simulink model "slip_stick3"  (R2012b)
settings: Solver=ode2  StartTime=0.0  StopTime=100  FixedStep=0.001  MaxStep=0.001  RelTol=1e-3
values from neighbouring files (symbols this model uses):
  c = 2200    [coulomb_1.m]    (also in coulomb_10.m = 0.1; coulomb_11.m = 0; coulomb_2.m; coulomb_3.m)
  FG = 500    [coulomb_1.m]    (also in coulomb_10.m = 10; coulomb_11.m = 10; coulomb_2.m; coulomb_3.m)
  FH = 12    [coulomb_10.m]    (also in coulomb_11.m; coulomb_3.m = 600; coulomb_4.m = 600; position_reg_1.m = 3.956)
  k = 10    [coulomb_10.m]    (also in coulomb_11.m; diff_filter_1.m = 250; diff_filter_2.m = 250; dry_friction_1.m = 2200)
  m = 400    [coulomb_1.m]    (also in coulomb_10.m = 10; coulomb_11.m = 10; coulomb_2.m; coulomb_3.m)
  vb = 0.1    [coulomb_10.m]    (also in coulomb_11.m; slip_stick_3.m; slip_stick_31.m; slip_stick_3_1.m)
  vs = 0.05    [position_reg_1.m]    (also in position_reg_2.m; slip_stick_21.m; slip_stick_3.m = 0.01; slip_stick_31.m)
undefined symbols (not defined in the file or in its folder): sgn

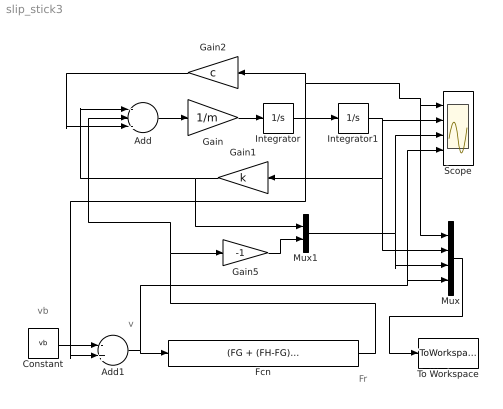
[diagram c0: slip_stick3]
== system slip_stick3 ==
  note: v
  note: vb
  note: Fr
  Add : Sum  Inputs=---
  Add1 : Sum  Inputs=-+
  Constant : Constant  Value=vb
  Fcn : Fcn  Expr=(FG + (FH-FG)*exp(-(u/vs)^2))*sgn(u)
  Gain : Gain  Gain=1/m
  Gain1 : Gain  Gain=k
  Gain2 : Gain  Gain=c
  Gain5 : Gain  Gain=-1
  Integrator : Integrator
  Integrator1 : Integrator
  Mux : Mux
  Mux1 : Mux  Inputs=2
  Scope : Scope  NumInputPorts=4
  To Workspace : ToWorkspace  VariableName=y  SampleTime=-1  SaveFormat=Structure With Time
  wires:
  Add/1 -> Gain/1
  Gain/1 -> Integrator/1
  Integrator1/1 -> Mux/2, Gain1/1, Scope/2
  Constant/1 -> Add1/1
  Integrator/1 -> Add1/2, Integrator1/1, Gain2/1, Mux/1, Scope/1
  Fcn/1 -> Add/2, Gain5/1
  Gain1/1 -> Mux1/1, Add/1
  Mux1/1 -> Mux/3, Scope/3
  Gain5/1 -> Mux1/2
  Add1/1 -> Mux/4, Scope/4, Fcn/1
  Mux/1 -> To Workspace/1
  Gain2/1 -> Add/3
